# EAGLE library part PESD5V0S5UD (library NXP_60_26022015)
Fivefold ESD protection diode arrays Fivefold ElectroStatic Discharge (ESD) protection diode arrays in a SOT457 (SC-74) small Surface-Mounted Device (SMD) plastic package designed to protect up to ﬁve signal lines from the damage caused by ESD and other transients. AAL Eindhoven MK
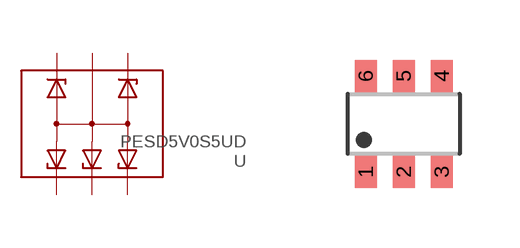
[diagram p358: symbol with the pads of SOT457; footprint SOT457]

Designator prefix U

## PESD5V0S5UD  [SOT457]
1  K1  pas
2  CA  pas
3  K2  pas
4  K3  pas
5  K4  pas
6  K5  pas

## Footprint SOT457 (pad centres in mm)
SOT457 TSOP6: Plastic surface-mounted package; 6 lead JEIDA: SC73 A.K.A. SOT23-6
smd 0.55 x 0.8: 1 -0.95,-1.2; 2 0,-1.2; 3 0.95,-1.2; 4 0.95,1.2; 5 0,1.2; 6 -0.95,1.2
